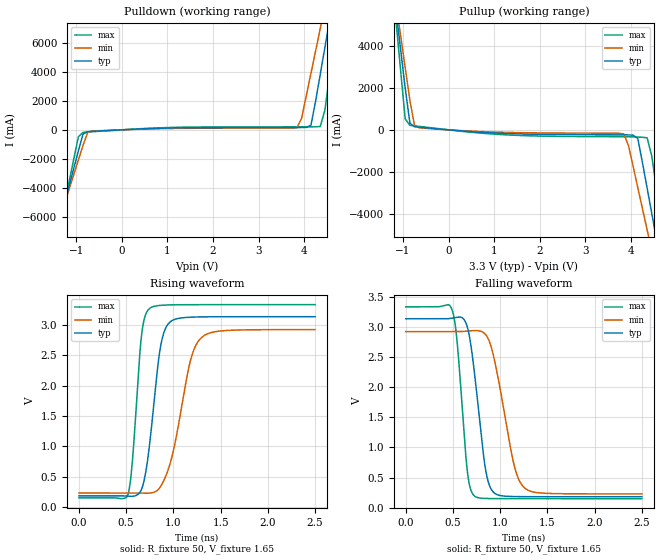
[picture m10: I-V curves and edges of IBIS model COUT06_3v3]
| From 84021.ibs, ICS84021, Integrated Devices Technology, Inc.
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[Model] COUT06_3v3
Model_type   Output
Polarity   Non-Inverting
|   typ   min   max
C_comp   2pF   1.5pF   2.5pF
Vmeas = 1.65V
Rref = 50
Vref = 1.65V
|   typ   min   max
[Voltage range]   3.3V   3.135V   3.465V
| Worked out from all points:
|   slope of the pulldown table from 0 to 0.495 V, typ, clamps not added: 6.88 ohm
|   slope of the pullup table from 0 to 0.495 V, typ, clamps not added: 5.83 ohm
|   rising waveform, R_fixture 50, V_fixture 1.65: 20-80 % time 127ps typ, 201ps min, 86.3ps max; typ from 0.181 V to 3.14 V
|   falling waveform, R_fixture 50, V_fixture 1.65: 20-80 % time 128ps typ, 189ps min, 92.7ps max; typ from 3.14 V to 0.181 V
[pulldown]
|Voltage   I (typ)   I (min)   I (max)
-3.3V     -29.26A    -25.24A    -35.98A
-1.463V   -7.508A    -7.113A    -8.217A
-1.361V   -6.298A    -6.106A    -6.67A
-952.6mV  -1.454A    -2.076A    -481.7mA
-850.5mV  -293.8mA   -1.069A    -175.5mA
-646.4mV  -102mA     -81.18mA   -129.6mA
3.844V    159mA      144.7mA    203.8mA
4.151V    319.9mA    3.884A     206.6mA
4.355V    3.815A     6.961A     228.9mA
4.559V    7.514A     10.04A     3.725A
4.763V    11.22A     13.12A     8.46A
6.6V      44.81A     41.05A     51.4A
[pullup]
|Voltage   I (typ)   I (min)   I (max)
-3.3V     44.73A     38.54A     55.09A
-1.157V   5.7A       6.046A     5.224A
-1.055V   3.84A      4.498A     2.846A
-952.6mV  1.979A     2.95A      516.9mA
-850.5mV  318.6mA    1.402A     214.1mA
-748.5mV  147.6mA    205.9mA    188.2mA
3.844V    -239.7mA   -193.2mA   -328.3mA
4.151V    -416.1mA   -2.755A    -342.5mA
4.355V    -2.772A    -4.758A    -379.9mA
4.559V    -5.183A    -6.764A    -2.792A
4.763V    -7.594A    -8.771A    -5.873A
6.6V      -29.3A     -26.85A    -33.6A
[Ramp]
|   typ   min   max
dV/dt_r   2.374/0.197n   2.162/0.318n   2.564/0.133n
dV/dt_f   2.390/0.193n   2.173/0.283n   2.581/0.140n
[Rising Waveform]
R_fixture = 50
V_fixture = 1.65
V_fixture_max = 1.7325
V_fixture_min = 1.56
C_fixture = 0.0p
| Time   typ   min   max
0s        180.7mV    228.1mV    148.5mV
517.1ps   175.7mV    228.2mV    190.5mV
564.8ps   172.8mV    228.4mV    725.4mV
662.6ps   287.2mV    227.2mV    2.825V
748ps     1.026V     225.5mV    3.276V
863.4ps   2.637V     331.6mV    3.328V
971.4ps   3.061V     746.1mV    3.336V
1.175ns   3.132V     2.376V     3.339V
1.298ns   3.137V     2.795V     3.339V
2.5ns     3.141V     2.927V     3.339V
[Falling Waveform]
R_fixture = 50
V_fixture = 1.65
V_fixture_max = 1.7325
V_fixture_min = 1.56
C_fixture = 0.0p
| Time   typ   min   max
0s        3.141V     2.927V     3.339V
489.5ps   3.152V     2.927V     3.292V
542.2ps   3.165V     2.927V     2.783V
652.6ps   2.999V     2.936V     592.4mV
727.9ps   2.231V     2.945V     192.6mV
828.3ps   806.2mV    2.905V     153.4mV
888.5ps   358.5mV    2.748V     150.6mV
1.142ns   184.2mV    738.8mV    148.6mV
1.252ns   181.9mV    336.5mV    148.5mV
2.5ns     180.7mV    228.1mV    148.5mV
